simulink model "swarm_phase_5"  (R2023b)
settings: Solver=ode3  StartTime=0.0  StopTime=t_end  FixedStep=dt8dof  RelTol=1e-3
PreLoadFcn:
  | define_swarm_buses(3, 1000);
model workspace (MAT data in the model file):
  L_wb = 2.8
  d_max = 0.558505360638
  dt8dof = 0.002
  dtastar = 0.1
  dtcontrol = 0.03
  gear_ratio = 10
  id1 = 1
  id2 = 2
  id3 = 3
  m_veh = 1300
  phi_road0_1 = 0.0285737917266
  phi_road0_2 = 0.0309082700445
  phi_road0_3 = 0.0327741623934
  psi0_1 = 0.610865238198
  psi0_2 = 0.610865238198
  psi0_3 = 0.610865238198
  r_wheel = 0.317
  slope_x_body0_1 = -0.0260871088594
  slope_x_body0_2 = -0.0282266776002
  slope_x_body0_3 = -0.0310980828185
  slope_y_body0_1 = 0.0285815707348
  slope_y_body0_2 = 0.0309181162484
  slope_y_body0_3 = 0.0327859021796
  t_end = 70
  teta0_1 = 0.0285737917266
  teta0_2 = 0.0309082700445
  teta0_3 = 0.0327741623934
  tetapunto0_1 = 0
  tetapunto0_2 = 0
  tetapunto0_3 = 0
  theta_road0_1 = -0.0260811935248
  theta_road0_2 = -0.0282191846907
  theta_road0_3 = -0.031088063742
  v_max_follower = 9.2
  v_max_leader = 8
  v_min = 0
  velstart_1 = 5
  velstart_2 = 5
  velstart_3 = 5
  wr0_FL_1 = 25.7731958763
  wr0_FL_2 = 25.7731958763
  wr0_FL_3 = 25.7731958763
  wr0_FR_1 = 25.7731958763
  wr0_FR_2 = 25.7731958763
  wr0_FR_3 = 25.7731958763
  wr0_RL_1 = 25.7731958763
  wr0_RL_2 = 25.7731958763
  wr0_RL_3 = 25.7731958763
  wr0_RR_1 = 25.7731958763
  wr0_RR_2 = 25.7731958763
  wr0_RR_3 = 25.7731958763
  x0_1 = 90
  x0_2 = 80
  x0_3 = 70
  y0_1 = 20
  y0_2 = 15
  y0_3 = 5

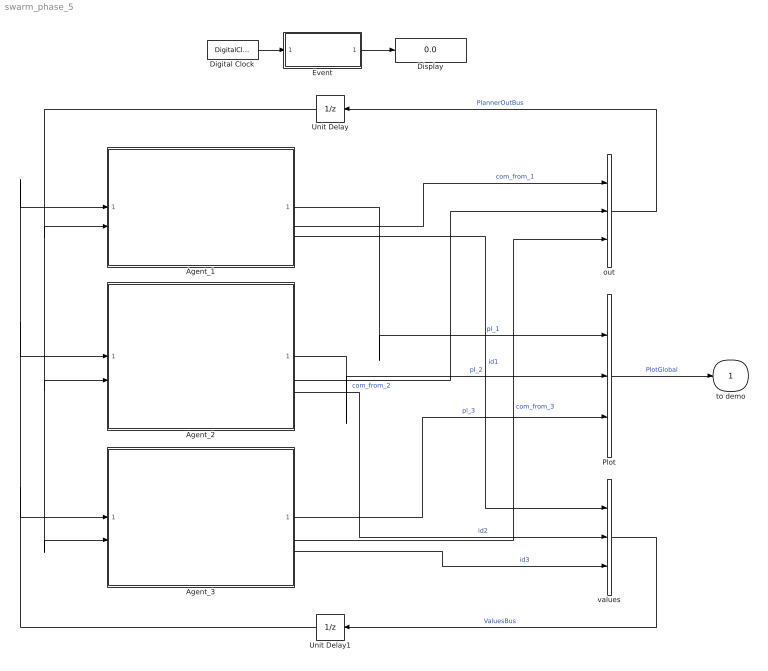
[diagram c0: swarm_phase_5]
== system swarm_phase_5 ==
  Agent_1 : ModelReference  ModelNameDialog=Agent.slx  UsingDefaultArgumentValue=0,0,0,0,0,0,0,0,0,0,0,0,0,0,0  SimulationMode=Normal  ModelReferenceVersion=1.99
  Agent_2 : ModelReference  ModelNameDialog=Agent.slx  UsingDefaultArgumentValue=0,0,0,0,0,0,0,0,0,0,0,0,0,0,0  SimulationMode=Normal  ModelReferenceVersion=1.99
  Agent_3 : ModelReference  ModelNameDialog=Agent.slx  UsingDefaultArgumentValue=0,0,0,0,0,0,0,0,0,0,0,0,0,0,0  SimulationMode=Normal  ModelReferenceVersion=1.99
  Digital Clock : DigitalClock  SampleTime=dtastar
  Display : Display
  Event : MATLAB Function  TreatAsAtomicUnit=on
  Plot : BusCreator  Inputs=3  OutDataTypeStr=Bus: PlotGlobal
  Unit Delay : UnitDelay  SampleTime=-1  HasFrameUpgradeWarning=on
  Unit Delay1 : UnitDelay  SampleTime=-1  HasFrameUpgradeWarning=on
  out : BusCreator  Inputs=3
  values : BusCreator  Inputs=3
  to demo : Outport  OutDataTypeStr=Bus: PlotGlobal  SampleTime=dtastar
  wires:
  Agent_1/1 -> Plot/1  "pl_1"
  Agent_2/1 -> Plot/2  "pl_2"
  Agent_3/1 -> Plot/3  "pl_3"
  Plot/1 -> to demo/1  "PlotGlobal"
  Agent_1/2 -> out/1  "com_from_1"
  Agent_2/2 -> out/2  "com_from_2"
  Agent_3/2 -> out/3  "com_from_3"
  out/1 -> Unit Delay/1  "PlannerOutBus"
  Agent_2/3 -> values/2  "id2"
  Agent_1/3 -> values/1  "id1"
  Unit Delay/1 -> Agent_2/2, Agent_3/2, Agent_1/2
  Agent_3/3 -> values/3  "id3"
  values/1 -> Unit Delay1/1  "ValuesBus"
  Unit Delay1/1 -> Agent_1/1, Agent_2/1, Agent_3/1
  Digital Clock/1 -> Event/1(t)
  Event/1(fired) -> Display/1

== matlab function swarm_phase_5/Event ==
function fired = MapEventInjector(t)
%#codegen
coder.extrinsic('apply_map_event');
fired = 0;
fired = apply_map_event(t);
end
